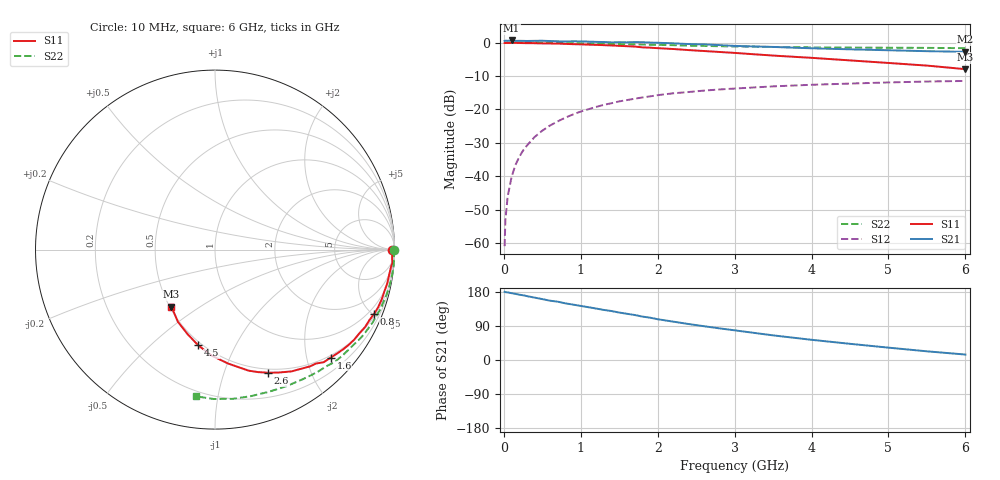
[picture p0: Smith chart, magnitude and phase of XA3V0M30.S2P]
! SIEMENS Discrete & RF Semiconductors
! BFY180
! Si NPN RF Bipolar Junction Transistor in MICRO-X
! VCE = 3 V  IC = 0.3 mA
! Common Emitter S-Parameters:  May  1997
# GHz  S  MA  R  50
!  f  S11  S21  S12  S22
! GHz  MAG  ANG  MAG  ANG  MAG  ANG  MAG  ANG
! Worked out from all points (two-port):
!   36 points, 10 MHz to 6 GHz, reference 50 ohm
!   highest |S21| = 0.63 dB at 100 MHz (marker M1); lowest = -2.8 dB at 6 GHz (marker M2)
!   |S21| within 3 dB of the highest: start of sweep to 5.123 GHz
!   lowest |S11| = -8.0 dB at 6 GHz (marker M3), VSWR 2.33, Z = 25.5 - j19.3 ohm
!   |S11| at or under -10 dB: nowhere
!   |S22| runs from -1.7 to 0.0 dB; largest |S21 - S12| = 1.1
!   S11 on the Smith chart (normalised r, x): 10 MHz: open; 800 MHz: 0.61, -5.10; 1.6 GHz: 0.46, -2.47; 2.6 GHz: 0.46, -1.42; 4.5 GHz: 0.48, -0.72; 6 GHz: 0.51, -0.39
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0.01  0.9855 -0.2  1.058 180.0  0.0009 84.9  0.9994 -0.1
0.02  0.984 -0.5  1.069 179.1  0.0022 94.9  0.9999 -0.5
0.05  0.9878 -1.2  1.061 178.3  0.005 85.1  0.9983 -1.0
0.1  0.9878 -2.8  1.075 176.4  0.0097 88.9  0.9975 -2.1
0.15  0.9913 -4.3  1.059 174.5  0.0147 87.0  0.9994 -3.2
0.2  0.9858 -5.4  1.062 172.4  0.0194 86.0  0.9986 -4.2
0.25  0.9821 -7.2  1.06 170.8  0.0243 84.6  0.9992 -5.3
0.4  0.978 -11.1  1.061 164.6  0.0387 81.3  0.9972 -8.3
0.6  0.9696 -16.5  1.054 156.5  0.0574 76.3  0.9909 -12.5
0.7  0.9641 -19.5  1.045 153.9  0.0662 73.6  0.9887 -14.6
0.8  0.9563 -21.9  1.035 149.5  0.0754 71.8  0.9837 -16.7
0.9  0.9457 -24.5  1.046 146.2  0.0842 69.2  0.9813 -18.7
1.1  0.9303 -29.9  1.033 139.3  0.1006 64.8  0.9716 -22.7
1.6  0.8819 -43.0  1.008 122.0  0.1379 54.3  0.9449 -32.5
1.8  0.8478 -48.5  1.013 114.6  0.1509 50.3  0.932 -36.1
2.2  0.8011 -57.9  0.975 101.3  0.1741 42.7  0.9145 -43.2
2.6  0.7474 -66.6  0.94 89.2  0.1911 36.3  0.8907 -49.5
3.5  0.6387 -83.5  0.86 65.0  0.221 23.7  0.8587 -62.4
4  0.5908 -91.8  0.821 53.3  0.2336 17.6  0.847 -69.4
4.5  0.541 -100.0  0.792 42.7  0.2435 12.0  0.8407 -76.3
5.5  0.4522 -117.2  0.743 22.9  0.2612 1.3  0.8324 -90.5
6  0.4 -127.3  0.727 14.4  0.2666 -4.1  0.8244 -97.5
